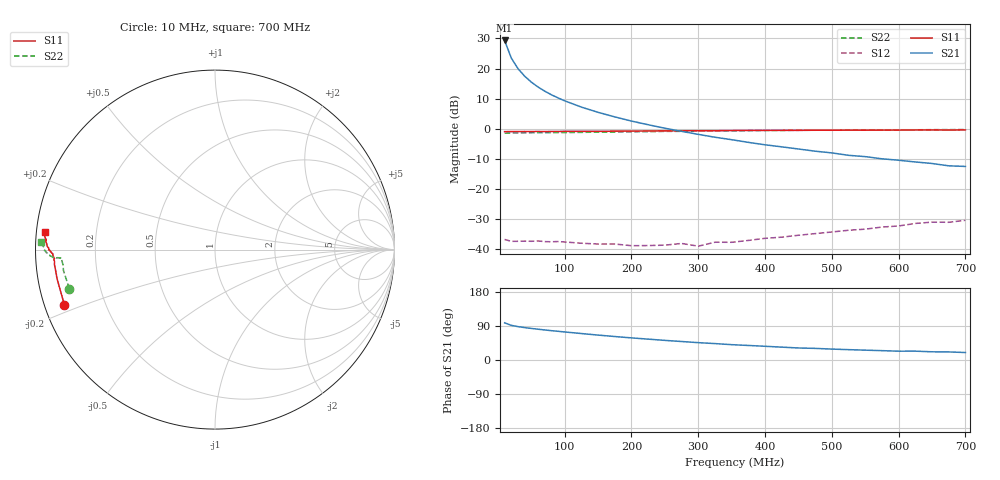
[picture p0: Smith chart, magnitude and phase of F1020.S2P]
! Date: Mon Aug 07 16:49:04 1995
# MHZ  S  MA  R  50.0000
!  POLYFET RF DEVICES
!  F1020 (Each Side)
!  S PARAMETERS
!  VDS=28V, IDQ=1.00A
!FREQ  S11MAG S11ANG S21MAG S21ANG S12MAG S12ANG S22MAG S22ANG
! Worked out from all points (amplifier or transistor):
!   34 points, 10 MHz to 700 MHz, reference 50 ohm
!   highest |S21| = 29.3 dB at 10 MHz (marker M1)
!   |S21| within 3 dB of that: start of sweep to 15.14 MHz
!   unconditionally stable (mu >= 1): 227.5 MHz to 398.1 MHz; 405.5 MHz to 428.8 MHz
!   at 60 MHz: K = 0.24, MSG = 25.6 dB, |S12| = -37.3 dB
!   at 300 MHz: K = 1.22, MAG = 15.8 dB, |S12| = -39.0 dB
!   at 700 MHz: K = 0.56, MSG = 9.0 dB, |S12| = -30.5 dB
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10  0.8936 -159.9  29.28 98.1  0.01443 12.1  0.8402 -164.9
20  0.8948 -169.4  14.94 91.4  0.01343 6.1  0.8523 -172.1
30  0.896 -173.1  9.961 88.1  0.01345 5.3  0.8508 -174.4
40  0.8986 -174.7  7.458 85.5  0.01356 3.7  0.8544 -175.5
50  0.8964 -175.8  5.95 83.3  0.01345 3.4  0.8557 -176.2
60  0.8996 -176.6  4.931 81.2  0.01363 2.9  0.8578 -176.5
70  0.8951 -176.9  4.212 79.3  0.01329 4.3  0.8556 -176.6
80  0.9013 -177.2  3.667 77.4  0.01321 4.9  0.8604 -176.9
90  0.9008 -177.6  3.249 75.7  0.01333 6.5  0.8632 -176.8
100  0.9031 -177.8  2.907 74.0  0.01309 4.2  0.8621 -176.8
125  0.904 -178.3  2.285 69.8  0.0125 9.1  0.8687 -176.9
150  0.904 -178.5  1.871 65.7  0.0121 13.0  0.878 -177.1
175  0.9103 -178.8  1.57 61.9  0.01212 16.2  0.8822 -177.0
200  0.9133 -179.2  1.338 58.4  0.01136 17.9  0.8874 -176.9
250  0.921 -179.8  1.018 51.8  0.0116 29.7  0.9031 -177.3
275  0.9259 -179.8  0.9038 48.8  0.01239 34.4  0.9034 -177.2
300  0.9265 179.7  0.8046 45.8  0.01116 39.6  0.9133 -177.7
325  0.9266 179.4  0.7211 43.3  0.01298 42.9  0.9197 -177.8
375  0.9356 178.8  0.5929 38.4  0.01389 51.7  0.9285 -178.3
475  0.9434 177.3  0.423 30.7  0.01805 63.8  0.9424 -179.4
600  0.9484 175.8  0.2991 23.2  0.02417 70.9  0.9568 179.0
700  0.9543 174.3  0.2359 19.7  0.03002 71.9  0.9678 177.6
